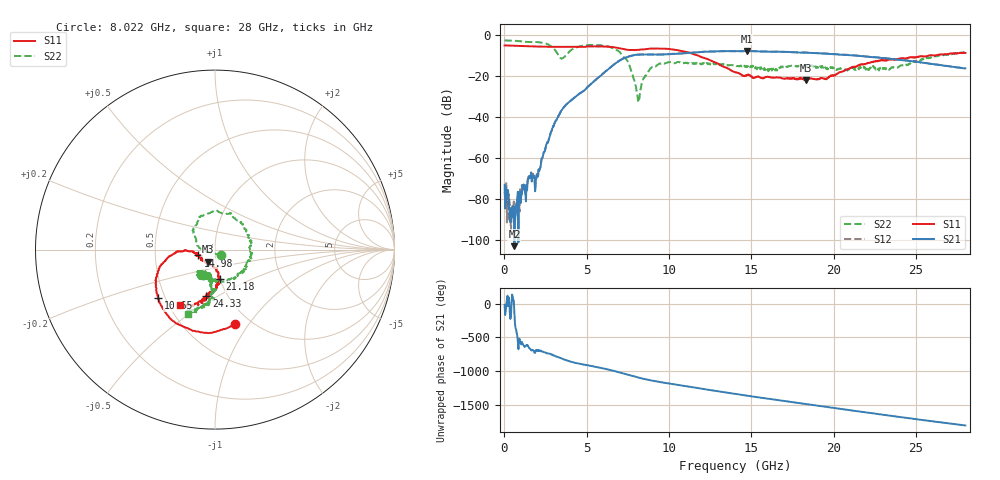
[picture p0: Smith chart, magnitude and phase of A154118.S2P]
!  2-Port S-parameters saved by WinCal
! VAR MeasName=S-Parameters (CALIBRATED_DATA) read from VNA (N5230A)
! VAR MeasDate=2015-9-10 14:34:33
! VAR NAME=A154118
! VAR FILENAME=A154118.S2P
! VAR DATE=2015-9-10 14:34:33
! VAR PHYS_PORTS=1,2
# Hz S DB R 50
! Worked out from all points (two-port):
!   801 points, 10 MHz to 28 GHz, reference 50 ohm
!   highest |S21| = -7.81 dB at 14.7 GHz (marker M1); lowest = -102.8 dB at 604.8 MHz (marker M2)
!   |S21| within 3 dB of the highest: 7.452 GHz to 22.42 GHz (14.96 GHz wide, 100 % of centre)
!   lowest |S11| = -22.1 dB at 18.31 GHz (marker M3), VSWR 1.17, Z = 45.8 - j6.27 ohm
!   |S11| at or under -10 dB: 11.75 GHz to 25.78 GHz (14.03 GHz wide, 74.8 % of centre); 26.12924 GHz to 26.15498 GHz (25.74 MHz wide, 0.0985 % of centre)
!   |S22| runs from -32.9 to -2.7 dB; largest |S21 - S12| = 0.008
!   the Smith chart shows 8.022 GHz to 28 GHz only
!   S11 on the Smith chart (normalised r, x): 8.022 GHz: 0.84, -0.86; 10.65 GHz: 0.46, -0.30; 14.98 GHz: 0.83, -0.05; 21.18 GHz: 1.00, -0.34; 24.33 GHz: 0.80, -0.45; 28 GHz: 0.57, -0.40
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1e7  -5.12 179.6  -72.91 -21.1  -76.46 -40.8  -2.67 179.8
6.047875e8  -5.25 162.4  -102.83 -143.9  -91.52 -78.9  -2.80 165.2
2.004288e9  -5.62 124.4  -68.75 20.3  -69.84 22.7  -3.47 127.6
2.66905e9  -5.72 104.6  -51.61 -19.4  -51.51 -21.7  -4.67 91.1
3.193862e9  -5.73 87.7  -40.96 -65.7  -40.90 -66.0  -8.70 25.6
3.753662e9  -5.76 68.6  -33.89 -118.8  -33.88 -118.5  -9.82 -108.6
4.698325e9  -5.82 33.6  -27.83 -178.1  -27.81 -178.1  -5.30 166.6
5.852912e9  -5.59 -11.6  -19.79 128.9  -19.76 129.2  -4.97 118.2
6.937525e9  -6.42 -52.6  -12.75 64.9  -12.67 64.8  -7.90 60.9
7.532312e9  -7.25 -66.7  -10.59 24.2  -10.52 24.0  -13.72 22.0
8.022138e9  -7.32 -75.3  -9.63 -8.3  -9.57 -8.5  -27.12 -39.6
9.351662e9  -6.63 -107.1  -9.57 -76.8  -9.46 -77.0  -14.19 118.6
1.06462e10  -7.62 -139.4  -9.08 -128.2  -8.98 -128.7  -13.37 64.4
1.4005e10  -18.10 -175.6  -7.90 104.5  -7.90 103.9  -14.91 -79.9
1.470475e10  -19.56 -166.3  -7.81 79.4  -7.77 78.9  -15.66 -89.1
1.498465e10  -20.21 -160.6  -7.85 69.2  -7.84 68.5  -15.02 -96.2
1.830846e10  -22.05 -120.4  -8.58 -46.0  -8.54 -46.1  -15.57 -113.4
1.869332e10  -21.22 -114.0  -8.71 -58.8  -8.74 -59.3  -14.72 -117.0
2.117744e10  -15.48 -80.2  -9.90 -142.9  -9.89 -143.6  -15.93 -113.5
2.334666e10  -12.01 -97.1  -11.50 144.5  -11.42 143.7  -16.82 -103.3
2.432631e10  -11.55 -100.7  -12.36 112.7  -12.31 112.0  -14.88 -95.4
2.8e10  -8.76 -122.8  -16.30 -2.2  -16.34 -3.2  -8.26 -112.8
